| TEXAS INSTRUMENTS INCORPORATED
| Standard Linear and Logic Group
| IBIS Model of SN74LVC2244A
| OCTAL BUFFER/DRIVER WITH 3-STATE OUTPUTS
| This file contains package information for the following:
|  TSSOP 20-pin (PW) package as [Component] LVC2244A_PW
|  SOIC 20-pin (DW) package as [Component] LVC2244A_DW
|  SSOP 20-pin (DB) package as [Component] LVC2244A_DB
|  SOP 20-pin (NS) package as [Component] LVC2244A_NS
|  TVSOP 20-pin (DGV) package as [Component] LVC2244A_DGV
| This device can be powered at the following Vccs:
|  1.8 volt Vcc
|  2.5 volt Vcc
|  3.3 volt Vcc
| This file provides unique models under the [Model Selector] for each Vcc.
| For operation at a specific Vcc, select the appropriate model after each
| [Model Selector] keyword.
[IBIS Ver]   3.2
[Comment char]  |_char
[File Name]   sn74lvc2244a.ibs
[File Rev]   1.1 | e_die
[Date]   April 12, 2002
[Source]   Data created from TI-SPICE simulations at TI-SLL.
[Notes]   The following is an IBIS list for the LVC2244A.
   Please contact sllibis@ti.com with questions and
   comments concerning SLL IBIS models.
   This IBIS model is created from a BA (back annotated netlist
   Non-montonic data in pullup due to over voltage tolerant
   C_comp values are taken at a different test condition
   than the data sheet.
[Disclaimer] Property of Texas Instruments Incorporated.  Unauthorized
   reproduction and/or distribution is strictly prohibited.
   This product is protected under copyright law.
   Created  2002, (C) Copyright  2002, Texas Instruments
   Incorporated, All Rights Reserved
   UNLESS THERE IS A SIGNED, WRITTEN AGREEMENT TO THE
   CONTRARY, TEXAS INSTRUMENTS (TI) IS PROVIDING THE IBIS
   MODELS  AND WITHOUT ANY WARRANTY, EXPRESSED OR
   IMPLIED.  TI assumes no liability for:
   1) the accuracy of the IBIS models provided to your
   company;
   2) the proper functioning of these IBIS Models in your
   design or for any resulting applications; or
   3) infringement of patents, copyrights or intellectual
   property rights resulting from your use of these IBIS
   models.
   TI provides IBIS Models as a service to our customers.
   You and your company shall not distribute, sell or give
   these models to anyone else without prior written
   permission from TI.
   TI reserves the right to make changes to our products or
   to discontinue any semiconductor product or service
   without notice, and advises our customers to obtain the
   latest version of relevant information to verify, before
   placing orders, that the information being relied on is
   current.
   Please be aware that your receipt and use of the IBIS
   information provided shall serve as acceptance of these
   terms and conditions.  If you do not accept these terms,
   you should return or destroy the IBIS models and any
   other accompanying information immediately.
| Component LVC2244A_PW 20-pin TSSOP
[Component]   LVC2244A_PW
[Manufacturer]   Texas Instruments, Inc.
[Package]
|   typ   min   max
R_pkg   4.500e-02   3.600e-02   5.700e-02
L_pkg   2.694e-09   2.290e-09   3.177e-09
C_pkg   1.560e-13   7.600e-14   2.590e-13
[Pin]   signal_name   model_name   R_pin   L_pin   C_pin
1   1NOE   LVC2244A_NOE   3.600e-02   3.045e-09   2.590e-13
2   1A1   LVC2244A_IN   5.100e-02   3.013e-09   1.890e-13
3   2Y4   LVC2244A_OUT   4.400e-02   2.695e-09   1.640e-13
4   1A2   LVC2244A_IN   4.700e-02   2.362e-09   7.900e-14
5   2Y3   LVC2244A_OUT   4.700e-02   2.333e-09   8.600e-14
6   1A3   LVC2244A_IN   4.700e-02   2.298e-09   8.500e-14
7   2Y2   LVC2244A_OUT   4.700e-02   2.351e-09   7.900e-14
8   1A4   LVC2244A_IN   4.400e-02   2.706e-09   1.650e-13
9   2Y1   LVC2244A_OUT   4.900e-02   2.999e-09   1.880e-13
10   GND   GND   3.900e-02   3.039e-09   2.570e-13
11   2A1   LVC2244A_IN   3.800e-02   3.044e-09   2.580e-13
12   1Y4   LVC2244A_OUT   5.700e-02   3.177e-09   1.990e-13
13   2A2   LVC2244A_IN   4.400e-02   2.825e-09   1.730e-13
14   1Y3   LVC2244A_OUT   4.700e-02   2.429e-09   8.300e-14
15   2A3   LVC2244A_IN   4.900e-02   2.383e-09   9.000e-14
16   1Y2   LVC2244A_OUT   4.900e-02   2.347e-09   8.900e-14
17   2A4   LVC2244A_IN   4.700e-02   2.290e-09   7.600e-14
18   1Y1   LVC2244A_OUT   4.500e-02   2.613e-09   1.580e-13
19   2NOE   LVC2244A_NOE   4.400e-02   2.883e-09   1.810e-13
20   VCC   POWER   3.900e-02   3.044e-09   2.560e-13
| Component LVC2244A_DW 20-pin SOIC
[Component]   LVC2244A_DW
[Manufacturer]   Texas Instruments, Inc.
[Package]
|   typ   min   max
R_pkg   3.800e-02   3.300e-02   4.500e-02
L_pkg   5.012e-09   4.110e-09   6.349e-09
C_pkg   7.170e-13   5.300e-13   8.680e-13
[Pin]   signal_name   model_name   R_pin   L_pin   C_pin
1   1NOE   LVC2244A_NOE   4.200e-02   6.336e-09   8.650e-13
2   1A1   LVC2244A_IN   4.300e-02   5.542e-09   8.670e-13
3   2Y4   LVC2244A_OUT   3.400e-02   4.714e-09   7.320e-13
4   1A2   LVC2244A_IN   3.400e-02   4.377e-09   5.910e-13
5   2Y3   LVC2244A_OUT   3.600e-02   4.130e-09   5.330e-13
6   1A3   LVC2244A_IN   3.500e-02   4.111e-09   5.300e-13
7   2Y2   LVC2244A_OUT   3.400e-02   4.284e-09   5.830e-13
8   1A4   LVC2244A_IN   3.400e-02   4.634e-09   7.260e-13
9   2Y1   LVC2244A_OUT   4.000e-02   5.518e-09   8.650e-13
10   GND   GND   4.300e-02   6.349e-09   8.660e-13
11   2A1   LVC2244A_IN   4.100e-02   6.281e-09   8.610e-13
12   1Y4   LVC2244A_OUT   4.500e-02   5.561e-09   8.680e-13
13   2A2   LVC2244A_IN   3.300e-02   4.778e-09   7.420e-13
14   1Y3   LVC2244A_OUT   3.500e-02   4.414e-09   5.960e-13
15   2A3   LVC2244A_IN   3.500e-02   4.110e-09   5.330e-13
16   1Y2   LVC2244A_OUT   3.600e-02   4.130e-09   5.330e-13
17   2A4   LVC2244A_IN   3.400e-02   4.377e-09   5.910e-13
18   1Y1   LVC2244A_OUT   3.400e-02   4.714e-09   7.310e-13
19   2NOE   LVC2244A_NOE   4.300e-02   5.569e-09   8.680e-13
20   VCC   POWER   4.200e-02   6.308e-09   8.640e-13
| Component LVC2244A_DB 20-pin SSOP
[Component]   LVC2244A_DB
[Manufacturer]   Texas Instruments, Inc.
[Package]
|   typ   min   max
R_pkg   4.000e-02   3.500e-02   5.100e-02
L_pkg   3.495e-09   3.035e-09   4.314e-09
C_pkg   4.200e-13   3.460e-13   5.020e-13
[Pin]   signal_name   model_name   R_pin   L_pin   C_pin
1   1NOE   LVC2244A_NOE   4.900e-02   4.310e-09   5.020e-13
2   1A1   LVC2244A_IN   4.800e-02   3.903e-09   4.870e-13
3   2Y4   LVC2244A_OUT   3.500e-02   3.189e-09   3.960e-13
4   1A2   LVC2244A_IN   3.500e-02   3.036e-09   3.470e-13
5   2Y3   LVC2244A_OUT   3.500e-02   3.035e-09   3.670e-13
6   1A3   LVC2244A_IN   3.500e-02   3.035e-09   3.670e-13
7   2Y2   LVC2244A_OUT   3.500e-02   3.036e-09   3.470e-13
8   1A4   LVC2244A_IN   3.500e-02   3.189e-09   3.970e-13
9   2Y1   LVC2244A_OUT   4.700e-02   3.899e-09   4.880e-13
10   GND   GND   5.100e-02   4.314e-09   5.000e-13
11   2A1   LVC2244A_IN   5.100e-02   4.314e-09   5.000e-13
12   1Y4   LVC2244A_OUT   4.700e-02   3.899e-09   4.880e-13
13   2A2   LVC2244A_IN   3.500e-02   3.189e-09   3.970e-13
14   1Y3   LVC2244A_OUT   3.500e-02   3.036e-09   3.460e-13
15   2A3   LVC2244A_IN   3.500e-02   3.035e-09   3.670e-13
16   1Y2   LVC2244A_OUT   3.500e-02   3.035e-09   3.670e-13
17   2A4   LVC2244A_IN   3.500e-02   3.036e-09   3.460e-13
18   1Y1   LVC2244A_OUT   3.500e-02   3.189e-09   3.970e-13
19   2NOE   LVC2244A_NOE   4.700e-02   3.899e-09   4.880e-13
20   VCC   POWER   5.100e-02   4.314e-09   5.020e-13
| Component LVC2244A_NS 20-pin SOP
[Component]   LVC2244A_NS
[Manufacturer]   Texas Instruments, Inc.
[Package]
|   typ   min   max
R_pkg   4.400e-02   2.900e-02   5.800e-02
L_pkg   3.666e-09   2.317e-09   5.115e-09
C_pkg   5.480e-13   3.160e-13   7.250e-13
[Pin]   signal_name   model_name   R_pin   L_pin   C_pin
1   1NOE   LVC2244A_NOE   5.800e-02   5.115e-09   7.250e-13
2   1A1   LVC2244A_IN   5.300e-02   4.591e-09   7.240e-13
3   2Y4   LVC2244A_OUT   4.900e-02   3.754e-09   5.720e-13
4   1A2   LVC2244A_IN   2.900e-02   2.549e-09   3.880e-13
5   2Y3   LVC2244A_OUT   3.100e-02   2.317e-09   3.160e-13
6   1A3   LVC2244A_IN   3.100e-02   2.317e-09   3.160e-13
7   2Y2   LVC2244A_OUT   2.900e-02   2.556e-09   3.990e-13
8   1A4   LVC2244A_IN   4.900e-02   3.754e-09   5.790e-13
9   2Y1   LVC2244A_OUT   5.300e-02   4.591e-09   7.240e-13
10   GND   GND   5.800e-02   5.115e-09   7.250e-13
11   2A1   LVC2244A_IN   5.800e-02   5.115e-09   7.250e-13
12   1Y4   LVC2244A_OUT   5.300e-02   4.591e-09   7.240e-13
13   2A2   LVC2244A_IN   4.900e-02   3.754e-09   5.790e-13
14   1Y3   LVC2244A_OUT   2.900e-02   2.557e-09   3.990e-13
15   2A3   LVC2244A_IN   3.100e-02   2.317e-09   3.160e-13
16   1Y2   LVC2244A_OUT   3.100e-02   2.317e-09   3.160e-13
17   2A4   LVC2244A_IN   2.900e-02   2.557e-09   3.990e-13
18   1Y1   LVC2244A_OUT   4.900e-02   3.754e-09   5.790e-13
19   2NOE   LVC2244A_NOE   5.300e-02   4.591e-09   7.240e-13
20   VCC   POWER   5.800e-02   5.115e-09   7.250e-13
| Component LVC2244A_DGV 20-pin TVSOP
[Component]   LVC2244A_DGV
[Manufacturer]   Texas Instruments, Inc.
[Package]
|   typ   min   max
R_pkg   4.400e-02   3.800e-02   4.800e-02
L_pkg   2.561e-09   2.236e-09   2.961e-09
C_pkg   3.420e-13   2.640e-13   4.460e-13
[Pin]   signal_name   model_name   R_pin   L_pin   C_pin
1   1NOE   LVC2244A_NOE   4.400e-02   2.935e-09   4.170e-13
2   1A1   LVC2244A_IN   4.200e-02   2.869e-09   4.460e-13
3   2Y4   LVC2244A_OUT   4.300e-02   2.399e-09   3.160e-13
4   1A2   LVC2244A_IN   4.400e-02   2.236e-09   2.650e-13
5   2Y3   LVC2244A_OUT   4.600e-02   2.278e-09   2.640e-13
6   1A3   LVC2244A_IN   4.500e-02   2.274e-09   2.640e-13
7   2Y2   LVC2244A_OUT   4.400e-02   2.285e-09   2.690e-13
8   1A4   LVC2244A_IN   4.300e-02   2.452e-09   3.200e-13
9   2Y1   LVC2244A_OUT   4.400e-02   2.900e-09   4.460e-13
10   GND   GND   4.400e-02   2.961e-09   4.180e-13
11   2A1   LVC2244A_IN   4.500e-02   2.954e-09   4.180e-13
12   1Y4   LVC2244A_OUT   4.200e-02   2.847e-09   4.430e-13
13   2A2   LVC2244A_IN   4.500e-02   2.453e-09   3.190e-13
14   1Y3   LVC2244A_OUT   4.500e-02   2.297e-09   2.690e-13
15   2A3   LVC2244A_IN   4.800e-02   2.334e-09   2.680e-13
16   1Y2   LVC2244A_OUT   4.800e-02   2.335e-09   2.670e-13
17   2A4   LVC2244A_IN   4.600e-02   2.299e-09   2.680e-13
18   1Y1   LVC2244A_OUT   4.600e-02   2.457e-09   3.200e-13
19   2NOE   LVC2244A_NOE   4.300e-02   2.848e-09   4.410e-13
20   VCC   POWER   3.800e-02   2.812e-09   4.080e-13
| Model LVC2244A_IN
[Model Selector]   LVC2244A_IN
LVC2244A_IN_18   1.8 volt Vcc
LVC2244A_IN_25   2.5 volt Vcc
LVC2244A_IN_33   3.3 volt Vcc
| Model LVC2244A_NOE
[Model Selector]   LVC2244A_NOE
LVC2244A_NOE_18   1.8 volt Vcc
LVC2244A_NOE_25   2.5 volt Vcc
LVC2244A_NOE_33   3.3 volt Vcc
| Model LVC2244A_OUT
[Model Selector]   LVC2244A_OUT
LVC2244A_OUT_18   1.8 volt Vcc
LVC2244A_OUT_25   2.5 volt Vcc
LVC2244A_OUT_33   3.3 volt Vcc
| Models and submodels in the file (9): LVC2244A_IN_18 (Input), LVC2244A_IN_25 (Input), LVC2244A_IN_33 (Input), LVC2244A_NOE_18 (Input), LVC2244A_NOE_25 (Input), LVC2244A_NOE_33 (Input), LVC2244A_OUT_18 (3-state), LVC2244A_OUT_25 (3-state), LVC2244A_OUT_33 (3-state)
